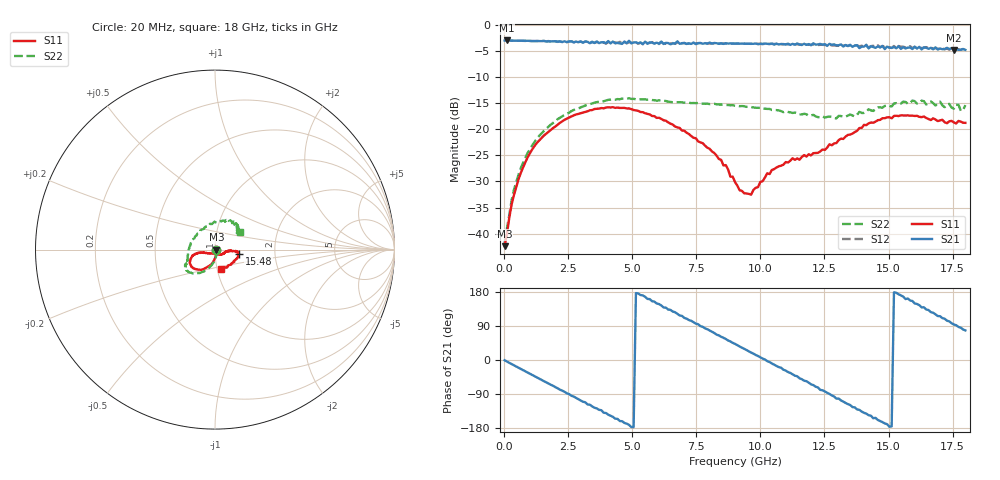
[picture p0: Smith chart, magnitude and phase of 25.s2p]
!Agilent Technologies,N5230A,US43500223,A.07.50.48
!Agilent N5230A: A.07.50.48
!Date: Tuesday, January 12, 2016 15:43:24
!Correction: S11(Full 2 Port(1,2))
!S21(Full 2 Port(1,2))
!S12(Full 2 Port(1,2))
!S22(Full 2 Port(1,2))
!S2P File: Measurements: S11, S21, S12, S22:
# Hz S  dB  R 50
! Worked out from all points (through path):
!   201 points, 20 MHz to 18 GHz, reference 50 ohm
!   highest |S21| = -3.01 dB at 109.9 MHz (marker M1); lowest = -4.8 dB at 17.55 GHz (marker M2)
!   group delay of S21, straight-line fit = 98.8 ps
!   lowest |S11| = -42.4 dB at 20 MHz (marker M3), VSWR 1.02, Z = 50.8 - j0.0726 ohm
!   |S11| at or under -10 dB: start of sweep to end of sweep
!   |S22| runs from -41.8 to -14.1 dB; largest |S21 - S12| = 0.042
!   S11 on the Smith chart (normalised r, x): 20 MHz: 1.02, -0.00; 15.48 GHz: 1.31, -0.06; 18 GHz: 1.04, -0.23
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2e7  -42.38 -5.4  -3.01 -0.7  -3.01 -0.9  -41.76 -3.9
1.099e8  -40.02 -33.5  -3.01 -4.1  -3.03 -4.2  -39.01 -32.1
5.594e8  -29.64 -80.1  -3.06 -20.2  -3.06 -20.3  -28.74 -79.7
1.0988e9  -23.85 -96.9  -3.12 -39.5  -3.12 -39.6  -23.06 -95.7
2.1776e9  -18.79 -116.9  -3.18 -78.1  -3.19 -78.2  -17.80 -115.1
3.0766e9  -16.81 -129.1  -3.44 -110.1  -3.38 -110.0  -15.65 -126.8
3.7958e9  -15.94 -139.2  -3.35 -132.6  -3.48 -133.5  -14.69 -135.3
4.515e9  -15.92 -148.5  -3.56 -161.1  -3.27 -160.9  -14.26 -142.4
5.5039e9  -16.94 -159.7  -3.23 166.7  -3.47 167.0  -14.29 -149.4
6.0433e9  -17.80 -166.0  -3.62 147.7  -3.69 146.4  -14.47 -151.9
7.3918e9  -21.63 -168.8  -3.39 99.8  -3.49 99.6  -14.98 -153.6
8.0211e9  -23.74 -163.1  -3.41 77.7  -3.58 77.1  -15.19 -154.5
9.01e9  -30.10 -133.5  -3.62 42.6  -3.60 41.8  -15.49 -157.0
9.6393e9  -32.52 -85.9  -3.66 19.6  -3.63 19.5  -15.77 -160.6
1.04484e10  -27.80 -43.3  -3.59 -9.2  -3.66 -9.5  -16.32 -169.0
1.20666e10  -24.58 -14.2  -3.54 -66.2  -3.77 -67.7  -17.25 156.2
1.3505e10  -21.00 -4.6  -3.83 -118.9  -3.92 -119.1  -17.18 112.5
1.50333e10  -17.70 -6.2  -4.40 -176.0  -4.30 -176.1  -15.55 70.1
1.54828e10  -17.35 -10.1  -4.63 170.6  -4.19 167.9  -15.11 63.9
1.66515e10  -18.24 -31.3  -4.42 126.4  -4.32 125.4  -14.69 46.4
1.75505e10  -18.69 -58.4  -4.84 93.7  -4.71 91.6  -16.08 38.6
1.8e10  -18.78 -74.2  -4.81 78.0  -4.85 75.7  -15.40 34.8
